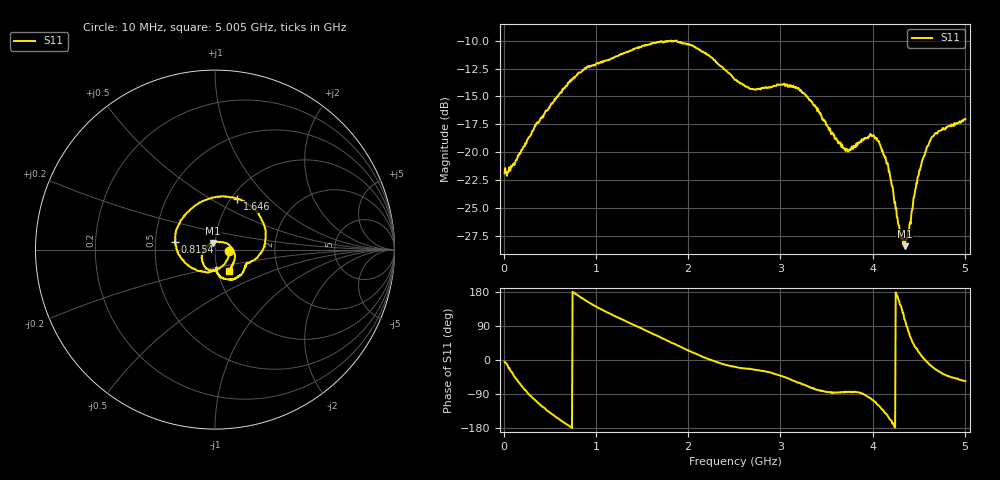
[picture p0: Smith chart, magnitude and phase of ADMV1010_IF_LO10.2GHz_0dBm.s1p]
! Analog Devices, Inc.
! 1 Analog Way
! Wilmington, MA 01887
! http://www.analog.com
! Date:  2021-09-07 NN
! Board Name:  ADMV1010-EVALZ Revision B with ADMV1010AEZ installed
! File Description:  S-Parameters for evaluation board without connectors or board loss de-embedded
! File Generation:  Calibrated Network Analyzer
! Chip Part Number:  ADMV1010
! Chip Description:  GaAs, MMIC, IQ Downconverter
! Chip Frequency:  12.6 to 15.4 GHz
! Chip Package:  LCC, 4.9 x 4.9 x 1 mm
! Chip State:
!  Temperature:  25C
!  LO Frequency:  10.2GHz
!  LO Power:  0dBm
! Note:
!  Analog Devices supplies this data as a sample of measured data at the evaluation board
!  ports for this product.  Your particular data for this product may vary.
!  Analog Devices reserves the right to change this data at anytime.
!  All lines below in this file are as is from the Network Analyzer.
!Keysight Technologies,N5245A,MY49151104,A.10.65.16
!Date: Thursday, August 05, 2021 16:36:10
!Correction: S22(Full 2 Port(1,2))
!S1P File: Measurement: S22:
# Hz S  dB  R 50
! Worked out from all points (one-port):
!   801 points, 10 MHz to 5.005 GHz, reference 50 ohm
!   lowest |S11| = -28.4 dB at 4.349 GHz (marker M1), VSWR 1.08, Z = 48.9 + j3.57 ohm
!   |S11| at or under -10 dB: start of sweep to 1.812 GHz; 1.816 GHz to 1.871 GHz (55.33 MHz wide, 3 % of centre); 1.878 GHz to end of sweep
!   S11 on the Smith chart (normalised r, x): 10 MHz: 1.17, -0.02; 815.4 MHz: 0.63, +0.06; 1.646 GHz: 1.07, +0.67; 5.005 GHz: 1.14, -0.27
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1e7  -21.89 -4.6
1.223875e8  -21.00 -45.9
3.34675e8  -17.75 -104.1
6.34375e8  -14.44 -161.7
8.154438e8  -12.85 168.7
9.965125e8  -12.11 141.7
1.25875e9  -11.29 109.9
1.452306e9  -10.63 87.9
1.645862e9  -10.20 66.1
1.883125e9  -10.12 38.4
2.145362e9  -10.95 9.7
2.5075e9  -13.53 -18.3
2.701056e9  -14.33 -24.8
3.131875e9  -14.12 -53.8
3.437819e9  -16.65 -80.1
3.612644e9  -18.92 -86.2
3.75625e9  -19.70 -84.4
3.987269e9  -18.56 -103.5
4.05595e9  -18.97 -118.3
4.162094e9  -20.99 -146.9
4.286969e9  -26.57 155.3
4.324431e9  -27.65 124.2
4.349406e9  -28.43 105.8
4.380625e9  -27.33 81.6
4.486769e9  -22.24 25.7
4.611644e9  -19.16 -10.7
4.699056e9  -18.35 -27.1
5.005e9  -17.04 -56.1
